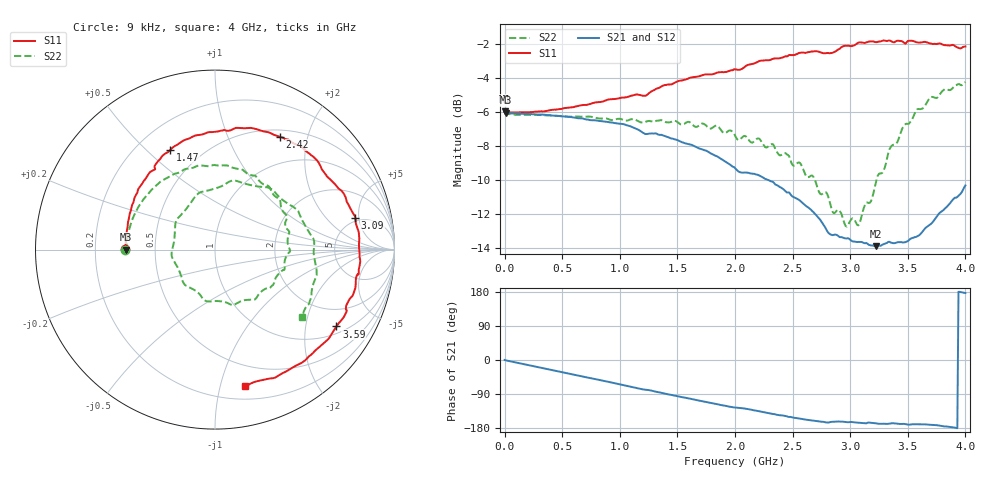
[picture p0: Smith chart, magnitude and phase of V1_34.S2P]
! ZVRE, 3.40
! symbol freq-unit parameter-type data-format keyword impedance-ohm
#  HZ  S  RI  R  50
! freq  reS11  imS11  reS21  imS21  reS12  imS12  reS22  imS22
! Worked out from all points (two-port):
!   401 points, 9 kHz to 4 GHz, reference 50 ohm
!   highest |S21| = -5.98 dB at 9 kHz (marker M1); lowest = -13.9 dB at 3.22 GHz (marker M2)
!   |S21| within 3 dB of the highest: start of sweep to 1.929 GHz
!   lowest |S11| = -6.1 dB at 10.01 MHz (marker M3), VSWR 2.98, Z = 16.8 + j0.0135 ohm
!   |S11| at or under -10 dB: nowhere
!   |S22| runs from -12.7 to -4.2 dB; largest |S21 - S12| = 0.0082
!   S11 on the Smith chart (normalised r, x): 9 kHz: 0.33, +0.00; 1.47 GHz: 0.34, +0.59; 2.42 GHz: 0.59, +1.57; 3.09 GHz: 4.50, +4.47; 3.59 GHz: 1.25, -2.97; 4 GHz: 0.31, -1.19
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9000  -0.5001 0.00123  0.5022 0.000818  0.5021 -0.00133  -0.5003 -0.000634
1.000898e7  -0.4978 0.000304  0.4962 -0.00787  0.4985 -0.00272  -0.4931 0.00859
3.200083e8  -0.4897 0.1139  0.4601 -0.1738  0.4648 -0.1712  -0.4538 0.1852
6.700075e8  -0.4628 0.2454  0.3498 -0.3275  0.3556 -0.3252  -0.3321 0.3528
1.050007e9  -0.3877 0.394  0.1741 -0.4248  0.179 -0.4273  -0.1298 0.454
1.340006e9  -0.307 0.5028  0.0361 -0.4275  0.0387 -0.4316  0.0576 0.4689
1.470006e9  -0.2493 0.5548  -0.0264 -0.4157  -0.023 -0.418  0.1469 0.448
1.830005e9  -0.0527 0.6476  -0.161 -0.3355  -0.1607 -0.3371  0.3576 0.2826
2.000004e9  0.0531 0.6658  -0.198 -0.2794  -0.1964 -0.28  0.3957 0.1609
2.210004e9  0.1985 0.678  -0.2318 -0.2289  -0.2297 -0.2309  0.4178 -0.0109
2.420004e9  0.3632 0.6276  -0.2482 -0.1628  -0.2479 -0.1641  0.3298 -0.185
2.670003e9  0.5497 0.5155  -0.2401 -0.089  -0.2396 -0.0943  0.1018 -0.3092
2.800003e9  0.6184 0.417  -0.216 -0.0578  -0.2166 -0.0651  -0.0601 -0.2812
2.910002e9  0.688 0.3405  -0.2047 -0.064  -0.2072 -0.063  -0.1752 -0.1862
3.090002e9  0.7811 0.1782  -0.2015 -0.0512  -0.2021 -0.0542  -0.2246 0.0865
3.220002e9  0.8021 0.0336  -0.1965 -0.0463  -0.1983 -0.0514  -0.1191 0.2839
3.340001e9  0.8001 -0.1361  -0.2035 -0.0431  -0.2046 -0.0443  0.0815 0.3796
3.470001e9  0.7483 -0.2778  -0.2032 -0.0405  -0.2043 -0.0434  0.3031 0.3428
3.590001e9  0.6764 -0.4281  -0.213 -0.0393  -0.2167 -0.0419  0.4635 0.2152
3.690001e9  0.5925 -0.5326  -0.2302 -0.0371  -0.2338 -0.0381  0.546 0.0645
3.81e9  0.4455 -0.6496  -0.2569 -0.0224  -0.2585 -0.0231  0.5661 -0.127
4e9  0.1656 -0.7618  -0.304 0.0171  -0.3029 0.0197  0.4826 -0.3782
